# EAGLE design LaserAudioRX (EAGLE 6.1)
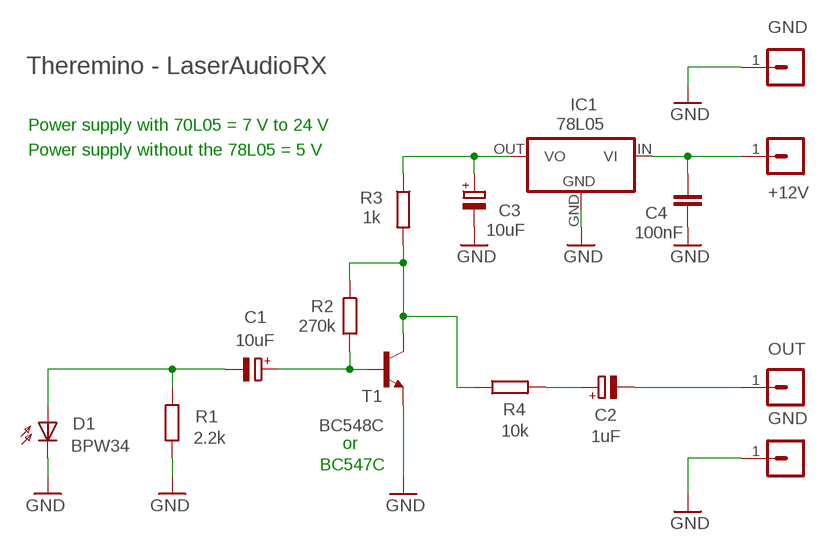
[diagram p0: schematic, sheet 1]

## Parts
C1  10uF  CPOL-EUE2-5B  [E2-5B]
C2  1uF  CPOL-EUE2-5B  [E2-5B]
C3  10uF  CPOL-EUE2-5B  [E2-5B]
C4  100nF  C-EU025-025X050  [C025-025X050]
D1  BPW34  [BPW34]
IC1  78L05  78REG  [TO92-REG]
R1  2.2k  R-EU_0204/5  [0204/5]
R2  270k  R-EU_0204/7  [0204/7]
R3  1k  R-EU_0204/7  [0204/7]
R4  10k  R-EU_0204/7  [0204/7]
SV1  GND  MA01-1  [MA01-1]
SV2  GND  MA01-1  [MA01-1]
SV3  OUT  MA01-1  [MA01-1]
SV4  +12V  MA01-1  [MA01-1]
T1  BC548C  -NPN-TO92-CBE  [TO92-CBE]

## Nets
GND: C3.V- C4.2 D1.K(C) IC1.GND R1.2 SV1.1 SV2.1 T1.E
N$1: R2.1 R3.2 R4.1 T1.C
N$2: C2.V+ R4.2
N$3: C4.1 IC1.IN(VI) SV4.1
N$4: C1.V+ R2.2 T1.B
N$5: C3.V+ IC1.OUT(VO) R3.1
N$6: C1.V- D1.A R1.1
N$7: C2.V- SV3.1

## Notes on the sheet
- Theremino - LaserAudioRX
- Power supply with 70L05 = 7 V to 24 V
- Power supply without the 78L05 = 5 V
- or
- BC547C

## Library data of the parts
C1-C3 = 00-LIVIO:CPOL-EU: POLARIZED CAPACITOR, European symbol
C4 = 00-LIVIO:C-EU: CAPACITOR, European symbol
D1 = 00-LIVIO:BPW34: PHOTO DIODE
IC1 = 00-LIVIO:78*: Positive VOLTAGE REGULATOR Source: http://cache.national.com/ds/LM/LM78L05.pdf http://www.fairchildsemi.com/ds/LM/LM7805.pdf
R1-R4 = 00-LIVIO:R-EU_: RESISTOR, European symbol
SV1-SV4 = 03-con-lstb-M:MA01-1: PIN HEADER
T1 = 00-LIVIO:*-NPN-: NPN Transistror

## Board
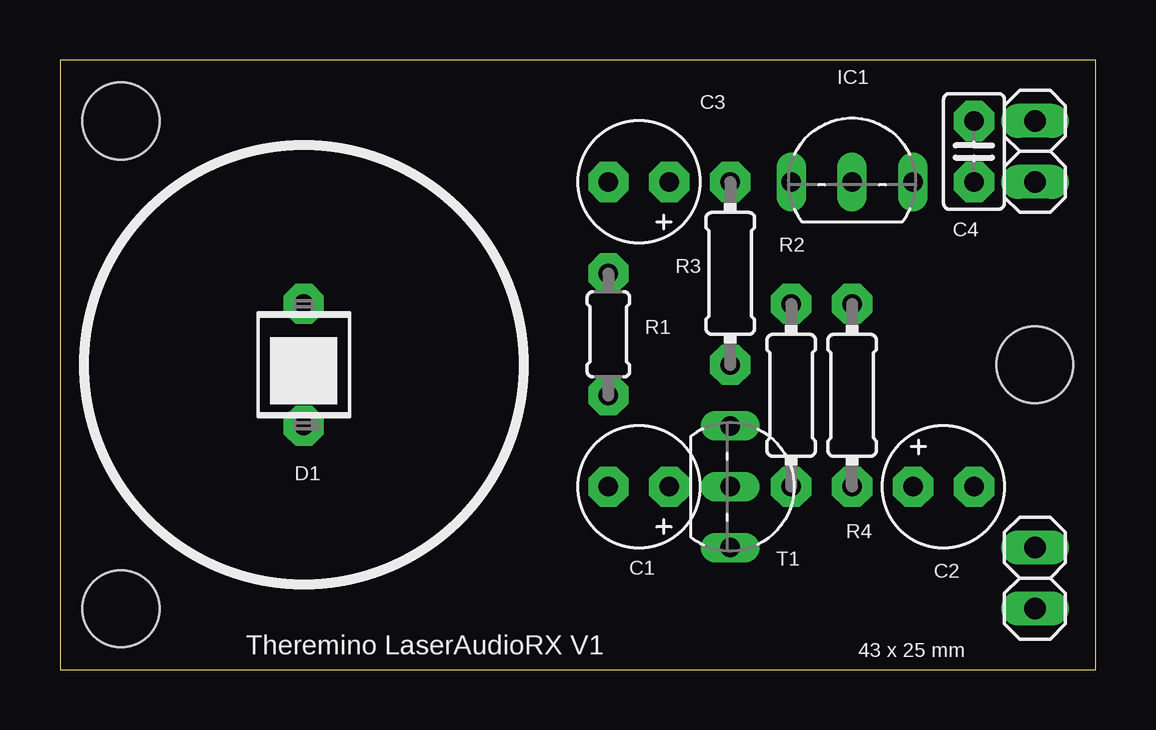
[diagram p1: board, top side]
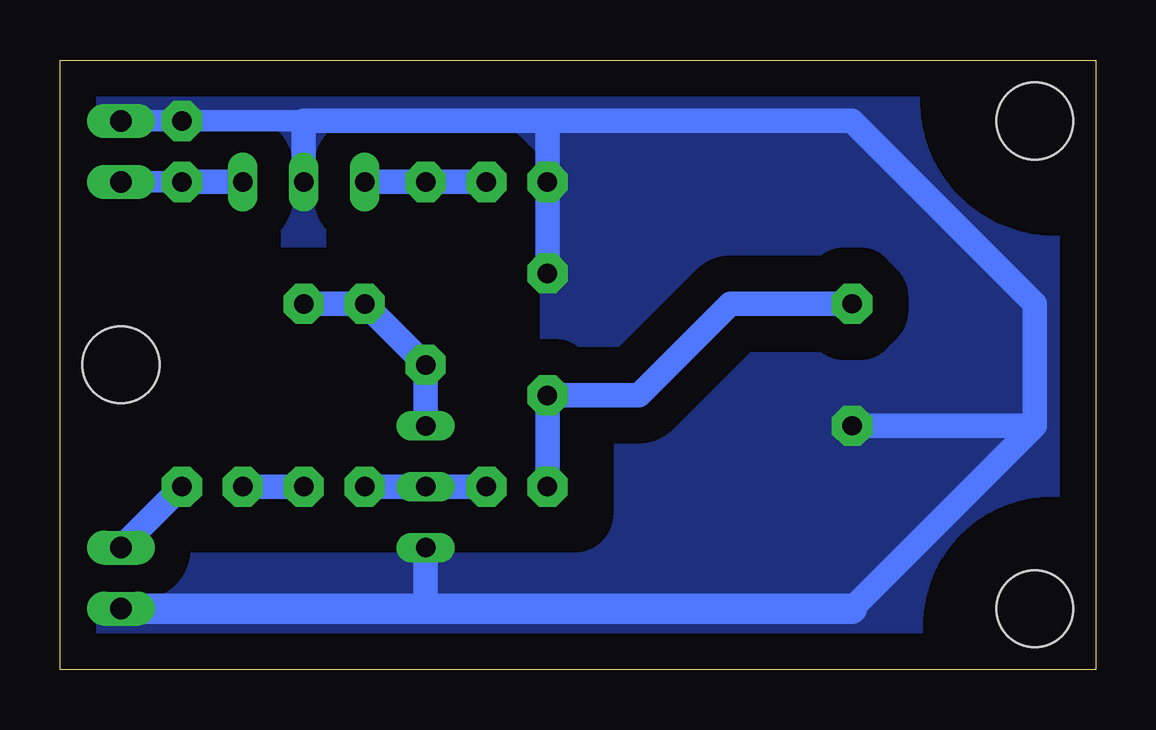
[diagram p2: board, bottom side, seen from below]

Size 43.18 x 25.4 mm. Coordinates in mm from the lower left corner, seen from the top.
Outline: 0,0 43.18,0 43.18,25.4 0,25.4 0,0
Copper layers (1*16): Top 0.035mm / dielectric 1.5mm / Bottom 0.035mm
Design rules: minimum track width 10mil, minimum drill 23mil, track to track 23mil, track to pad 23mil, pad to pad 23mil, via to via 23mil, smd to smd 23mil, copper to edge 23mil, drill to drill 8mil, minimum pad ring 5mil, minimum via ring 8mil, stop-mask expansion 4mil, vias tented up to drill 0mil, thermal gap 35mil
Holes 3.2 mm at 2.54,22.86 2.54,2.54 40.64,12.7
bRestrict: 5 lines

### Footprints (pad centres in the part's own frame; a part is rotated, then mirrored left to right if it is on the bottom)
E2-5B = drill 0.813 pad 1.676 octagon: V+ -1.27,0; V- 1.27,0
C025-025X050 = drill 0.813 pad 1.676 octagon: 1 -1.27,0; 2 1.27,0
BPW34 = drill 0.8 pad 1.676 octagon: A 0,2.54; K 0,-2.54
TO92-REG = drill 0.813 long: GND 0,0; IN 2.54,0; OUT -2.54,0
0204/5 = drill 0.813 pad 1.676 octagon: 1 -2.54,0; 2 2.54,0
0204/7 = drill 0.813 pad 1.676 octagon: 1 -3.81,0; 2 3.81,0
MA01-1 = drill 0.9 pad 1.422 long: 1 0,0
TO92-CBE = drill 0.813 long: B 0,0; C -2.54,0; E 2.54,0

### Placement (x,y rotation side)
C1  24.13,7.62 180 top
C2  36.83,7.62 0 top
C3  24.13,20.32 180 top
C4  38.1,21.59 90 top
D1  10.16,12.7 0 top
IC1  33.02,20.32 0 top
R1  22.86,13.97 90 top
R2  30.48,11.43 270 top
R3  27.94,16.51 270 top
R4  33.02,11.43 270 top
SV1  40.64,2.54 90 top
SV2  40.64,22.86 90 top
SV3  40.64,5.08 90 top
SV4  40.64,20.32 90 top
T1  27.94,7.62 270 top

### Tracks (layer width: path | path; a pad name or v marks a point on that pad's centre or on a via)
GND
  Bottom 0.9: 33.02,22.86 C4.2 SV2.1
  Bottom 1.016: 22.86,22.86 33.02,22.86 IC1.GND | 22.86,22.86 10.16,22.86 2.54,15.24 2.54,10.16 | 2.54,10.16 10.16,2.54 | R1.2 22.86,22.86 | D1.K 2.54,10.16 | T1.E 27.94,2.54
  Bottom 1.27: SV1.1 27.94,2.54 10.16,2.54
  pour Bottom (isolate 1.5, no thermals): -1,-1 44.18,-1 44.18,26.4 -1,26.4
N$1
  Bottom 1.016: R4.1 R2.1 R3.2 T1.C
N$2
  Bottom 1.016: R4.2 C2.V+
N$3
  Bottom 0.9: C4.1 SV4.1
  Bottom 1.016: C4.1 IC1.IN
N$4
  Bottom 1.016: C1.V+ T1.B R2.2
N$5
  Bottom 1.016: C3.V+ R3.1 IC1.OUT
N$6
  Bottom 1.016: C1.V- R1.1 19.05,11.43 15.24,15.24 D1.A
N$7
  Bottom 1.016: C2.V- SV3.1

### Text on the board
tNames: Theremino LaserAudioRX V1 | 43 x 25 mm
